|Texas Instruments Incorporated
|64 Channel Analog Front End for Digital X-Ray Detector
| Marketing part#   Digital Voltage Range   Package-type   #pins
|AFE0064IPBK   3.2V TO 3.6V   LQFP   128
|AFE0064IPBKR   3.2V TO 3.6V   LQFP   128
[IBIS Ver]   4.0
[File name]   afe0064.ibs
[File Rev]   1.0
[Date]   10/10/2010
[Source]   Texas Instruments Incorporated.
   Analog-eLab, HPA
   12500 TI Blvd
   Dallas, TX -75243
   For Support e-mail: elab_ibis@list.ti.com
[Notes]   Revision History:
   1.0: 10/10/2010
   - Initial version of the model
   - Initial Model generated from simulations in TISPICED
   - Model names with a trailing _33 contains the model for
   33V (3.2V and 3.4V).
   - Model not matched to measurements
   - C_comp although listed in numerical order of value are
   obtained from varying PVT conditions. For PVT conditions
   for each specific value refer the buffer description under
   respective [Model]. IBIS model user is responsible for using
   appropriate C_comp to simulate for Signal Integrity.
[Disclaimer]
 This product is designed as an aid for customers of Texas Instruments.
 No warranties, either expressed or implied, with respect to this third
 party software (if any) or with respect to its fitness for any
 particular purpose is claimed by Texas Instruments or the author. The
 software (if any) is provided solely on an "as is" basis. The entire
 risk as to its quality and performance is with the customer
[Copyright] (C) Copyright 2009 Texas Instruments Incorporated.
   All rights reserved.
|   AFE0064
[Component]   afe0064ipdb
[Manufacturer] TI
[Package]   | 128 LQFP - PBK package
| variable   typ   min   max
R_pkg  1.25766E-01   7.66000E-02   1.51180E-01
L_pkg  4.29251E+00nH  3.60812E+00nH  5.12685E+00nH
C_pkg  1.01600E+00pF  6.94820E-01pF  1.24874E+00pF
|-------------------------PIN------------------------------------------------
[Pin] signal_name  model_name  R_pin  L_pin C_pin
1   IN16   TERM   0.14697  5.11732nH  0.96734pF
2   IN17   TERM   0.14559  4.95204nH  1.23112pF
3   IN18   TERM   0.14468  4.85654nH  1.20673pF
4   IN19   TERM   0.14408  4.77824nH  1.18022pF
5   IN20   TERM   0.14375  4.71056nH  1.15316pF
6   IN21   TERM   0.14365  4.65037nH  1.12617pF
7   IN22   TERM   0.14376  4.59645nH  1.09959pF
8   IN23   TERM   0.14404  4.54875nH  1.07360pF
9   IN24   TERM   0.14449  4.50812nH  1.04816pF
10   IN25   TERM   0.14507  4.47737nH  1.02429pF
11   IN26   TERM   0.14605  4.48156nH  0.96322pF
12   IN27   TERM   0.14693  4.50413nH  0.93190pF
13   IN28   TERM   0.14804  4.53011nH  0.93147pF
14   IN29   TERM   0.14887  4.45419nH  0.88521pF
15   IN30   TERM   0.14992  4.44242nH  0.86953pF
16   IN31   TERM   0.15118  4.47635nH  0.74838pF
17   IN32   TERM   0.15118  4.47698nH  0.74749pF
18   IN33   TERM   0.14993  4.44390nH  0.86770pF
19   IN34   TERM   0.14886  4.45223nH  0.88168pF
20   IN35   TERM   0.14805  4.53277nH  0.93035pF
21   IN36   TERM   0.14694  4.50675nH  0.93134pF
22   IN37   TERM   0.14605  4.48448nH  0.96316pF
23   IN38   TERM   0.14508  4.48058nH  1.02495pF
24   IN39   TERM   0.14450  4.51169nH  1.04902pF
25   IN40   TERM   0.14406  4.55309nH  1.07464pF
26   IN41   TERM   0.14377  4.60141nH  1.10099pF
27   IN42   TERM   0.14367  4.65611nH  1.12753pF
28   IN43   TERM   0.14377  4.71709nH  1.15455pF
29   IN44   TERM   0.14411  4.78569nH  1.18179pF
30   IN45   TERM   0.14471  4.86442nH  1.20878pF
31   IN46   TERM   0.14562  4.96074nH  1.23306pF
32   IN47   TERM   0.14700  5.12685nH  0.96812pF
33   IN48   TERM   0.11914  4.59092nH  0.94167pF
34   IN49   TERM   0.11560  4.38454nH  1.20238pF
35   IN50   TERM   0.11273  4.25194nH  1.17416pF
36   IN51   TERM   0.11036  4.14014nH  1.14431pF
37   IN52   TERM   0.10842  4.04186nH  1.11430pF
38   IN53   TERM   0.10687  3.95397nH  1.08472pF
39   IN54   TERM   0.10568  3.87535nH  1.05587pF
40   IN55   TERM   0.10482  3.80575nH  1.02792pF
41   IN56   TERM   0.10428  3.74622nH  1.00080pF
42   IN57   TERM   0.10401  3.69907nH  0.97550pF
43   IN58   TERM   0.10427  3.68936nH  0.91326pF
44   IN59   TERM   0.10456  3.70053nH  0.88100pF
45   IN60   TERM   0.10522  3.71741nH  0.87985pF
46   IN61   TERM   0.10569  3.63449nH  0.83307pF
47   IN62   TERM   0.10651  3.61772nH  0.81707pF
48   IN63   TERM   0.10763  3.64875nH  0.69612pF
49   VSS   GND   0.10763  3.64928nH  0.69522pF
50   P_REF   TERM   0.10651  3.61870nH  0.81523pF
51   VSS   GND   0.10568  3.63173nH  0.82951pF
52   VSS   GND   0.10522  3.71887nH  0.87869pF
53   VDD   POWER   0.10457  3.70175nH  0.88039pF
54   VSS   GND   0.10428  3.69048nH  0.91314pF
55   VDD   POWER   0.10402  3.70018nH  0.97610pF
56   VT_A   TERM   0.10429  3.74739nH  1.00158pF
57   VT_B   TERM   0.10484  3.80739nH  1.02886pF
58   NC   NC   0.10570  3.87721nH  1.05716pF
59   VSS   GND   0.10689  3.95621nH  1.08595pF
60   VDD   POWER   0.10844  4.04449nH  1.11555pF
61   VDD   POWER   0.11039  4.14329nH  1.14573pF
62   VSS   GND   0.11276  4.25512nH  1.17605pF
63   STO   OBUF   0.11563  4.38814nH  1.20414pF
64   EOC   OBUF   0.11917  4.59475nH  0.94229pF
65   VSS   GND   0.14697  5.12302nH  0.96755pF
66   INTG   INBUF   0.14559  4.95714nH  1.23147pF
67   IRST   INBUF   0.14468  4.86124nH  1.20906pF
68   SHS   INBUF   0.07660  4.41025nH  1.24874pF
69   SHR   INBUF   0.07679  4.35771nH  1.23436pF
70   CLK   INBUF   0.07703  4.30984nH  1.20325pF
71   VSS   GND   0.14647  4.65205nH  1.11338pF
72   DF_SM   INBUF   0.14582  4.58585nH  1.08376pF
73   VSS   GND   0.14550  4.53022nH  1.05703pF
74   VSS   GND   0.14550  4.48777nH  1.03210pF
75   VDD   POWER   0.14605  4.48336nH  0.96703pF
76   VSS   GND   0.14693  4.50553nH  0.93213pF
77   OUTP_1   TERM   0.14804  4.53131nH  0.93154pF
78   OUTM_1   TERM   0.14887  4.45499nH  0.88525pF
79   VSS   GND   0.14992  4.44292nH  0.86955pF
80   VSS   GND   0.15118  4.47645nH  0.74839pF
81   VDD   POWER   0.15118  4.47688nH  0.74748pF
82   VSS   GND   0.14993  4.44340nH  0.86769pF
83   OUTM_0   TERM   0.14886  4.45143nH  0.88165pF
84   OUTP_0   TERM   0.14805  4.53157nH  0.93031pF
85   VSS   GND   0.14694  4.50535nH  0.93129pF
86   VSS   GND   0.14605  4.48268nH  0.96309pF
87   VDD   POWER   0.14508  4.47848nH  1.02488pF
88   PDZ   INBUF   0.14450  4.50929nH  1.04894pF
89   NAPZ   INBUF   0.14406  4.55039nH  1.07454pF
90   VSS   GND   0.14377  4.59831nH  1.10088pF
91   VSS   GND   0.14367  4.65261nH  1.12740pF
92   ENTRI   INBUF   0.14377  4.71319nH  1.15441pF
93   INTUPZ   INBUF   0.14411  4.78139nH  1.18163pF
94   PGA_2   INBUF   0.14471  4.85972nH  1.20861pF
95   PGA_1   INBUF   0.14562  4.95564nH  1.23287pF
96   PGA_0   INBUF   0.14700  5.12115nH  0.96797pF
97   STI   INBUF   0.11914  4.58462nH  0.94145pF
98   SMT_MD   INBUF   0.11560  4.37774nH  1.20209pF
99   VSS   GND   0.11273  4.24474nH  1.17386pF
100  VDD   POWER   0.11036  4.13264nH  1.14399pF
101  VSS   GND   0.10842  4.03406nH  1.11398pF
102  VSS   GND   0.10687  3.94587nH  1.08438pF
103  VSS   GND   0.10568  3.86695nH  1.05553pF
104  REFM   TERM   0.10482  3.79715nH  1.02756pF
105  REFP   TERM   0.10428  3.73732nH  1.00044pF
106  VDD   POWER   0.10401  3.68997nH  0.97513pF
107  VSS   GND   0.10427  3.68016nH  0.91288pF
108  VDD   POWER   0.10456  3.69113nH  0.88062pF
109  VSS   GND   0.10522  3.70791nH  0.87946pF
110  VSS   GND   0.10569  3.62489nH  0.83267pF
111  NC   NC   0.10651  3.60812nH  0.81668pF
112  EXT_C   TERM   0.10763  3.63905nH  0.69572pF
113  IN0   TERM   0.10763  3.63958nH  0.69482pF
114  IN1   TERM   0.10651  3.60910nH  0.81484pF
115  IN2   TERM   0.10568  3.62213nH  0.82911pF
116  IN3   TERM   0.10522  3.70937nH  0.87830pF
117  IN4   TERM   0.10457  3.69235nH  0.88001pF
118  IN5   TERM   0.10428  3.68128nH  0.91276pF
119  IN6   TERM   0.10402  3.69108nH  0.97572pF
120  IN7   TERM   0.10429  3.73849nH  1.00121pF
121  IN8   TERM   0.10484  3.79879nH  1.02850pF
122  IN9   TERM   0.10570  3.86881nH  1.05681pF
123  IN10   TERM   0.10689  3.94811nH  1.08561pF
124  IN11   TERM   0.10844  4.03669nH  1.11522pF
125  IN12   TERM   0.11039  4.13579nH  1.14541pF
126  IN13   TERM   0.11276  4.24792nH  1.17574pF
127  IN14   TERM   0.11563  4.38134nH  1.20384pF
128  IN15   TERM   0.11917  4.58845nH  0.94208pF
|   TERM Model
[Model] TERM
Model_type Terminator
|   typ   min   max
C_comp   1e-20   1e-20   1e-20
| variable   typ   min   max
[Voltage Range]   3.3V   3.2V   3.6V
[POWER Clamp Reference]  3.3V   3.2V   3.6V
[GND Clamp Reference]   0.0V   0.0V   0.0V
|Operating Temperature
[Temperature Range]   37   95   0
| Models and submodels in the file (3): TERM (Terminator), INBUF (Input), OBUF (Output)
